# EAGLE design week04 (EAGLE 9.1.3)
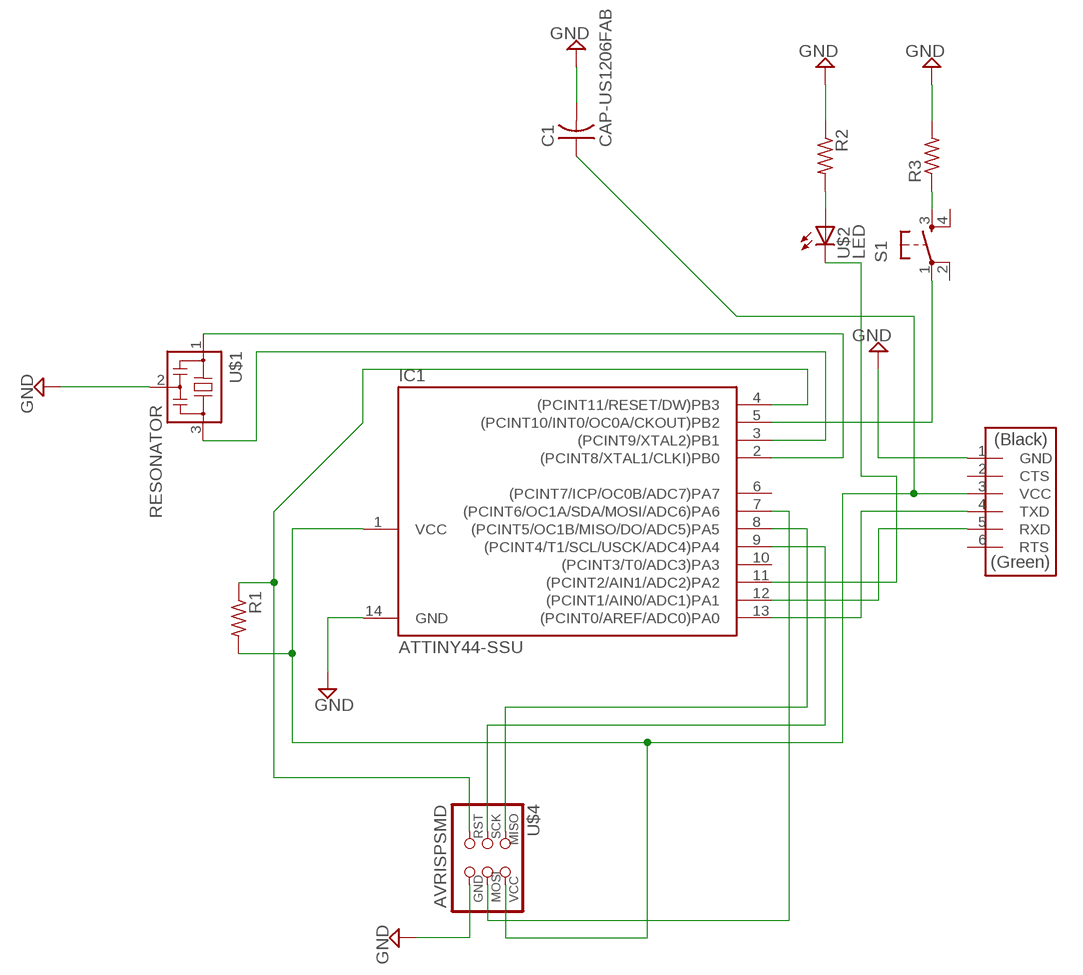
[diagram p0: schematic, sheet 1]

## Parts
C1  CAP-US1206FAB  [C1206FAB]
IC1  ATTINY44-SSU  [SOIC14]
R1  RES-US1206FAB  [R1206FAB]
R2  RES-US1206FAB  [R1206FAB]
R3  RES-US1206FAB  [R1206FAB]
S1  6MM_SWITCH6MM_SWITCH  [6MM_SWITCH]
U$1  RESONATOR  [EFOBM]
U$2  LED  [LED1206]
U$3  FTDI-SMD-HEADER  [1X06SMD]
U$4  AVRISPSMD  [2X03SMD]

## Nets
GND: C1.2 IC1.14(GND) R2.1 R3.2 U$1.2 U$3.1(GND) U$4.6(GND)
N$1: IC1.2((PCINT8/XTAL1/CLKI)PB0) U$1.1
N$2: IC1.3((PCINT9/XTAL2)PB1) U$1.3
N$3: C1.1 IC1.1(VCC) R1.2 U$3.3(VCC) U$4.2(VCC)
N$4: IC1.9((PCINT4/T1/SCL/USCK/ADC4)PA4) U$4.3(SCK)
N$5: IC1.8((PCINT5/OC1B/MISO/DO/ADC5)PA5) U$4.1(MISO)
N$6: IC1.4((PCINT11/RESET/DW)PB3) R1.1 U$4.5(RST)
N$7: IC1.7((PCINT6/OC1A/SDA/MOSI/ADC6)PA6) U$4.4(MOSI)
N$8: IC1.13((PCINT0/AREF/ADC0)PA0) U$3.4(TXD)
N$9: IC1.12((PCINT1/AIN0/ADC1)PA1) U$3.5(RXD)
N$10: R2.2 U$2.1(A)
N$11: IC1.11((PCINT2/AIN1/ADC2)PA2) U$2.2(C)
N$12: R3.1 S1.3(S)
N$13: IC1.5((PCINT10/INT0/OC0A/CKOUT)PB2) S1.1(P)
Unconnected: IC1.6((PCINT7/ICP/OC0B/ADC7)PA7) IC1.10((PCINT3/T0/ADC3)PA3) S1.2(P1) S1.4(S1) U$3.2(CTS) U$3.6(RTS)

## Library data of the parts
C1 = fab:CAP-US
IC1 = fab:ATTINY44
R1-R3 = fab:RES-US: Resistor (US Symbol)
S1 = fab:6MM_SWITCH: OMRON SWITCH
U$1 = fab:RESONATOR
U$2 = fab:LED: LED
U$3 = fab:FTDI-SMD-HEADER
U$4 = fab:AVRISP

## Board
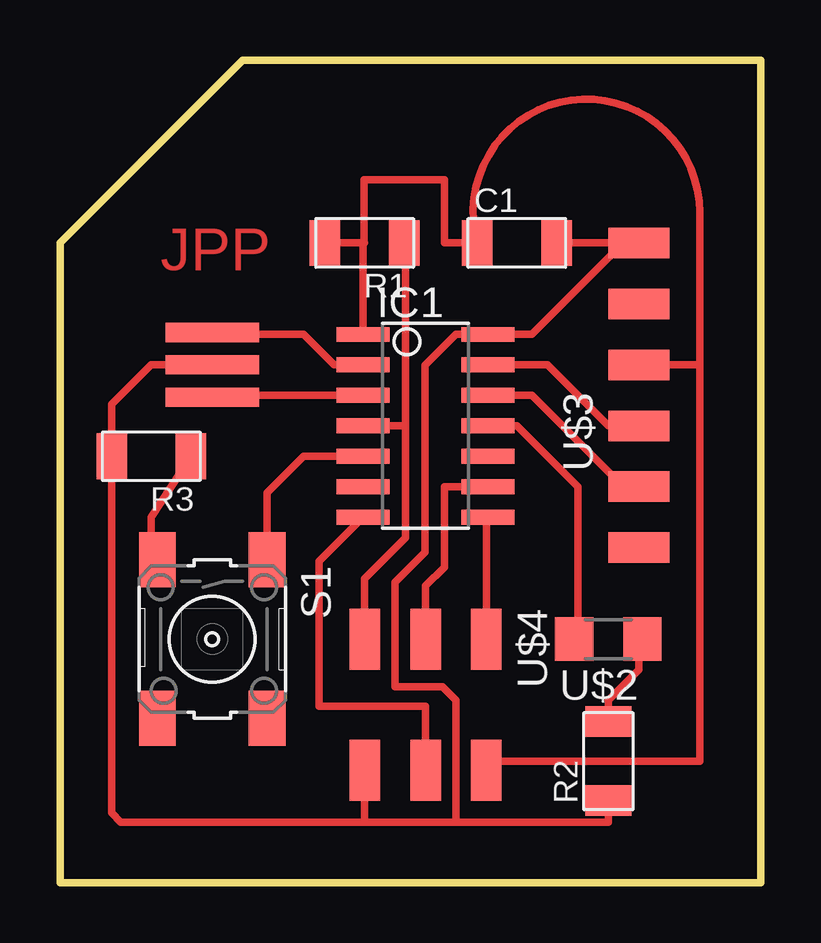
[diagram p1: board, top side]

Size 29.21 x 34.29 mm. Coordinates in mm from the lower left corner, seen from the top.
Outline: 0,0 0,26.67 7.62,34.29 29.21,34.29 29.21,0 0,0
Copper layers (1*16): Top 0.035mm / dielectric 1.5mm / Bottom 0.035mm
Design rules "default *": minimum track width 12mil, minimum drill 0.35mm, track to track 20mil, track to pad 20mil, pad to pad 20mil, via to via 20mil, smd to smd 20mil, copper to edge 40mil, drill to drill 6mil, minimum pad ring 10mil, minimum via ring 8mil, stop-mask expansion 4mil, vias tented up to drill 0mil, thermal gap 10mil

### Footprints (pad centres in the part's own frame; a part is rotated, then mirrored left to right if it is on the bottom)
C1206FAB = smd 1.27 x 1.905: 1 -1.651,0; 2 1.651,0
SOIC14 = smd 0.61 x 2.21: 1 -3.81,-2.603; 2 -2.54,-2.603; 3 -1.27,-2.603; 4 0,-2.603; 5 1.27,-2.603; 6 2.54,-2.603; 7 3.81,-2.603; 8 3.81,2.603; 9 2.54,2.603; 10 1.27,2.603; 11 0,2.603; 12 -1.27,2.603; 13 -2.54,2.603; 14 -3.81,2.603
R1206FAB = smd 1.27 x 1.905: 1 -1.651,0; 2 1.651,0
6MM_SWITCH = smd 2.286 x 1.524: 1 -3.302,2.286; 2 3.302,2.286; 3 -3.302,-2.286; 4 3.302,-2.286
EFOBM = smd 0.8 x 3.9: 1 -1.35,0; 2 0,0; 3 1.35,0
LED1206 = smd 1.6 x 1.803: 1 -1.422,0; 2 1.422,0
1X06SMD = smd 2.54 x 1.27: 1 0,6.35; 2 0,3.81; 3 0,1.27; 4 0,-1.27; 5 0,-3.81; 6 0,-6.35
2X03SMD = smd 2.54 x 1.27: 1 -2.54,2.54; 2 2.92,2.54; 3 -2.54,0; 4 2.92,0; 5 -2.54,-2.54; 6 2.92,-2.54

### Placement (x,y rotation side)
C1  19.05,26.67 0 top
IC1  15.24,19.05 270 top
R1  12.7,26.67 180 top
R2  22.86,5.08 90 top
R3  3.81,17.78 180 top
S1  6.35,10.16 270 top
U$1  6.35,21.59 270 top
U$2  22.86,10.16 180 top
U$3  24.13,20.32 0 top
U$4  15.24,7.62 270 top

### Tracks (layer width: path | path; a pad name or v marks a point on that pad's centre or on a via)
GND
  Top 0.305: U$1.2 3.81,21.59 2.16,19.94 R3.2 2.16,2.92 2.54,2.54 12.7,2.54 | R2.1 22.86,2.54 16.51,2.54 | 16.51,2.54 12.7,2.54 | U$4.6 12.7,2.54 | C1.2 U$3.1 23.49,26.67 19.68,22.86 IC1.14 16.51,22.86 15.21,21.57 15.21,13.77 13.97,12.53 13.97,8.18 15.95,8.18 16.51,7.62 16.51,2.54
N$1
  Top 0.305: U$1.1 6.35,22.86 10.16,22.86 11.43,21.59 IC1.2
N$2
  Top 0.305: U$1.3 6.43,20.32 IC1.3
N$3
  Top 0.305: U$4.2 17.78,5.08 26.67,5.08 26.67,21.59 | U$3.3 26.67,21.59 | 26.67,21.59 26.67,27.94 arc196 C1.1 16.03,26.67 16.03,29.3 12.68,29.3 12.68,26.69 12.7,26.67 12.64,26.67 | 12.64,26.67 R1.2 | IC1.1 12.64,26.67
N$4
  Top 0.305: IC1.9 16.03,16.51 16.03,13.16 15.24,12.37 U$4.3
N$5
  Top 0.305: U$4.1 17.78,15.24 IC1.8
N$6
  Top 0.305: U$4.5 12.7,12.68 14.4,14.39 14.4,19.05 | 14.4,19.05 14.4,26.62 R1.1 | IC1.4 14.15,19.05 14.4,19.05
N$7
  Top 0.305: IC1.7 10.79,13.4 10.79,7.37 15.24,7.37 U$4.4
N$8
  Top 0.305: IC1.13 20.32,21.59 22.86,19.05 U$3.4
N$9
  Top 0.305: IC1.12 19.68,20.32 23.49,16.51 U$3.5
N$10
  Top 0.305: 22.86,6.35 R2.2 22.86,7.62 24.13,8.89 24.13,10.16 U$2.1
N$11
  Top 0.305: IC1.11 19.05,19.05 21.59,16.51 21.59,10.16 U$2.2
N$12
  Top 0.305: S1.3 3.81,13.97 3.81,15.24 R3.1
N$13
  Top 0.305: IC1.5 10.16,17.78 8.64,16.26 S1.1

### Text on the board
Top: JPP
